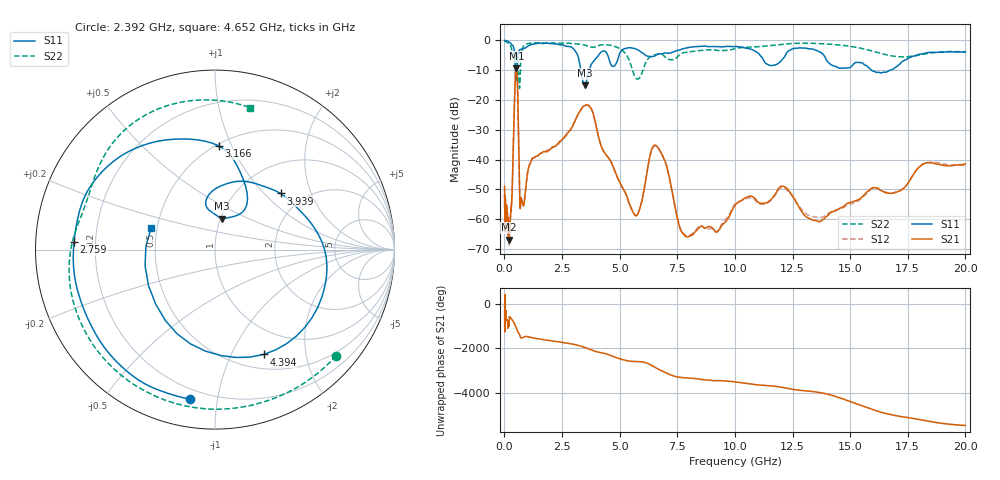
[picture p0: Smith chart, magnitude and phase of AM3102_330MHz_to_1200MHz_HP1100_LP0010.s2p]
! Date/Time: Tue, Sep 11, 2018 5:21 PM
! Network Analyzer: Agilent Technologies E8362B Rev: A.07.50.63
! Sweep from 0.010 to 20.000 GHz, 1601 Points, Sweep Type: LOG
! Power Supply: 4.949 V, 0.001 A
# Hz S DB R 50
!freq MagS11 AngS11 MagS21 AngS21 MagS12 AngS12 MagS22 AngS22
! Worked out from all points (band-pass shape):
!   1601 points, 10 MHz to 20 GHz, reference 50 ohm
!   highest |S21| = -9.39 dB at 520.6 MHz (marker M1); lowest = -66.8 dB at 182.2 MHz (marker M2)
!   |S21| within 3 dB of the highest: 475.5 MHz to 558.9 MHz (83.45 MHz wide, 16.1 % of centre)
!   lowest |S11| = -15.1 dB at 3.482 GHz (marker M3), VSWR 1.43, Z = 50.8 + j18 ohm
!   |S11| at or under -10 dB: 472.3 MHz to 534.4 MHz (62.14 MHz wide, 12.3 % of centre); 3.315 GHz to 3.678 GHz (363 MHz wide, 10.4 % of centre); 15.92 GHz to 16.76 GHz (841.6 MHz wide, 5.15 % of centre)
!   |S22| runs from -16.1 to -0.2 dB; largest |S21 - S12| = 0.0058
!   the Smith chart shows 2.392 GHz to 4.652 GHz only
!   S11 on the Smith chart (normalised r, x): 2.392 GHz: 0.14, -0.84; 2.759 GHz: 0.12, +0.03; 3.166 GHz: 0.51, +0.89; 3.939 GHz: 1.54, +1.25; 4.394 GHz: 0.67, -1.34; 4.652 GHz: 0.46, +0.13
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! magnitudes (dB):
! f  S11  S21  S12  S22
! 10 MHz  -0.1  -49.0  -51.7  -0.2
! 35.55 MHz  -0.1  -59.8  -58.3  -0.3
! 126.4 MHz  -0.3  -58.2  -59.6  -0.7
! 182.2 MHz  -0.5  -66.8  -64.9  -1.0
! 320.7 MHz  -1.5  -53.8  -53.6  -3.2
! 447.2 MHz  -4.5  -18.5  -18.5  -4.4
! 520.6 MHz  -10.8  -9.4  -9.4  -9.7
! 575.3 MHz  -6.5  -16.4  -16.5  -12.1
! 682.6 MHz  -3.1  -56.1  -56.5  -13.0
! 1.59 GHz  -1.0  -37.9  -37.8  -0.9
! 2.392 GHz  -1.5  -33.9  -34.4  -0.9
! 2.759 GHz  -2.1  -31.0  -31.3  -1.0
! 3.166 GHz  -4.8  -25.4  -25.4  -1.2
! 3.482 GHz  -15.1  -22.0  -21.9  -1.6
! 3.939 GHz  -6.4  -27.3  -27.3  -2.2
! 4.394 GHz  -3.8  -38.3  -38.2  -1.5
! 4.652 GHz  -8.5  -41.2  -41.3  -1.8
! 5.652 GHz  -2.8  -58.6  -58.5  -12.1
! 6.549 GHz  -5.2  -35.2  -35.4  -4.8
! 7.958 GHz  -2.5  -66.0  -65.7  -3.9
! 13.68 GHz  -3.9  -60.9  -59.4  -1.1
! 20 GHz  -3.9  -41.5  -42.0  -3.8
